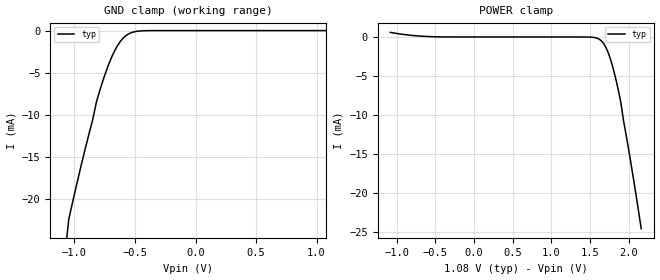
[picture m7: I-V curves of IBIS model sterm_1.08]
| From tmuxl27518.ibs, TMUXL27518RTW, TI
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| sterm_1.08
[Model]   sterm_1.08
Model_type   Terminator
|   typ   min   max
C_comp   1.598234e-12   NA   NA
[Voltage Range]   1.08   NA   NA
[Temperature Range]   27   NA   NA
[Power Clamp Reference]   1.08   NA   NA
[GND Clamp Reference]   0   NA   NA
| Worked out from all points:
|   GND clamp passes 1 mA (typ) near -0.60 V on its own axis
[GND Clamp]
|   Voltage   I(typ)   I(min)   I(max)
-2.16V    -123.9mA   NA         NA
-1.08V    -26.92mA   NA         NA
-1.047V   -22.42mA   NA         NA
-949.1mV  -16.28mA   NA         NA
-850.9mV  -10.67mA   NA         NA
-818.2mV  -8.452mA   NA         NA
-785.5mV  -6.864mA   NA         NA
-720mV    -4.102mA   NA         NA
-654.5mV  -2.029mA   NA         NA
-556.4mV  -414uA     NA         NA
-392.7mV  -7.228uA   NA         NA
1.08V     165.6pA    NA         NA
[POWER Clamp]
|   Voltage   I(typ)   I(min)   I(max)
-1.08V    586.7uA    NA         NA
-556.4mV  43.09uA    NA         NA
1.473V    -7.228uA   NA         NA
1.636V    -414uA     NA         NA
1.702V    -1.293mA   NA         NA
1.735V    -2.029mA   NA         NA
1.8V      -4.102mA   NA         NA
1.865V    -6.864mA   NA         NA
1.898V    -8.452mA   NA         NA
1.931V    -10.67mA   NA         NA
2.029V    -16.28mA   NA         NA
2.16V     -24.56mA   NA         NA
